(* Logix 5000 DataType export UDT_C30S_EnIP; software revision 20.01 *)

TYPE UDT_PLC2_to_30S :   // Output from PLC
STRUCT
   Automatic : BOOL;
   Start : BOOL;
   AckFault : BOOL;
   DS1 : BOOL;
   DS2 : BOOL;
   ExtDigSig : BOOL;
   Res1 : BOOL;
   Res2 : BOOL;
   Prog : SINT;
END_STRUCT
END_TYPE

TYPE UDT_C30S_to_PLC :   // Input to PLC
STRUCT
   NoFault : BOOL;
   ReadyToStart : BOOL;
   OK : BOOL;
   NOK : BOOL;
   DepthReached : BOOL;
   Res1 : BOOL;
   Res2 : BOOL;
   Res3 : BOOL;
   ProgResult : SINT;
   StrategyResult : SINT;
   CodeResult : INT;
   TorqueResult : REAL;
   PreTorqueResult : REAL;
   AngleResult : REAL;
   DepthResult : REAL;
   DriveTime : REAL;
   CycleNumber : DINT;
END_STRUCT
END_TYPE

TYPE UDT_C30S_EnIP :   // In and Output Data for Weber C30S
STRUCT
   OUT : UDT_PLC2_to_30S;   // Output Parameters
   IN : UDT_C30S_to_PLC;   // Input Parameters
END_STRUCT
END_TYPE
